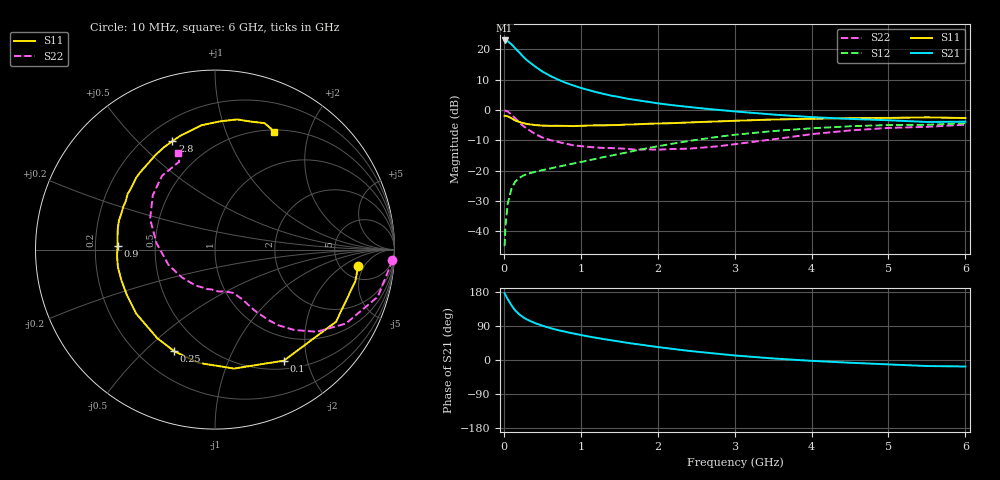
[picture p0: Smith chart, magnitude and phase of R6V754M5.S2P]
! SIEMENS Small Signal Semiconductors
! BFR193
! Si NPN RF Bipolar Junction Transistor in SOT23
! VCE = 0.75 V  IC = 4.5 mA
! Common Emitter S-Parameters:  May  1996
# GHz  S  MA  R  50
!  f  S11  S21  S12  S22
! GHz  MAG  ANG  MAG  ANG  MAG  ANG  MAG  ANG
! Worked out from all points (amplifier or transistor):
!   36 points, 10 MHz to 6 GHz, reference 50 ohm
!   highest |S21| = 22.9 dB at 10 MHz (marker M1)
!   |S21| within 3 dB of that: start of sweep to 164.5 MHz
!   unconditionally stable (mu >= 1): 883.6 MHz to 2.277 GHz
!   at 250 MHz: K = 0.41, MSG = 19.6 dB, |S12| = -21.6 dB
!   at 1.4 GHz: K = 1.09, MAG = 8.0 dB, |S12| = -15.0 dB
!   at 6 GHz: K = 1.00, MSG = 0.3 dB, |S12| = -4.4 dB
!   S11 on the Smith chart (normalised r, x): 10 MHz: 7.28, -3.67; 100 MHz: 0.62, -1.62; 250 MHz: 0.34, -0.62; 900 MHz: 0.30, +0.02; 2.8 GHz: 0.30, +0.64; 6 GHz: 0.52, +1.49
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0.01  0.8031 -6.4  14 176.3  0.0057 87.1  0.9891 -3.3
0.02  0.8016 -12.6  13.86 172.0  0.0117 85.6  0.975 -6.5
0.05  0.7851 -30.8  13.64 160.6  0.0285 75.1  0.9438 -16.2
0.1  0.728 -58.2  12.07 144.1  0.051 62.8  0.8374 -29.5
0.15  0.6712 -80.9  10.35 130.3  0.0666 53.6  0.7288 -38.9
0.2  0.6376 -98.3  8.914 120.6  0.0758 48.0  0.6277 -45.5
0.25  0.6099 -112.0  7.595 113.0  0.0829 44.5  0.5493 -50.1
0.3  0.5889 -123.2  6.628 106.9  0.0881 42.7  0.4944 -52.7
0.4  0.5658 -140.9  5.28 97.8  0.0952 41.0  0.4081 -56.8
0.5  0.5529 -152.2  4.317 90.5  0.102 41.2  0.3518 -59.3
0.6  0.549 -161.7  3.662 84.5  0.1087 42.2  0.3204 -60.9
0.7  0.5496 -169.6  3.195 79.1  0.1157 43.5  0.2983 -62.8
0.9  0.5434 177.9  2.546 70.1  0.1308 46.6  0.2627 -67.2
1.1  0.5546 167.5  2.134 62.1  0.1479 49.0  0.247 -73.0
1.3  0.5593 159.0  1.838 55.1  0.1677 50.6  0.2368 -78.9
1.6  0.5769 147.6  1.539 45.5  0.2003 51.7  0.2293 -90.2
2.2  0.6075 128.1  1.198 29.2  0.2793 49.3  0.2277 -118.1
2.8  0.6496 111.4  1.001 16.0  0.3634 42.3  0.2535 -152.0
3.5  0.6969 96.2  0.842 4.1  0.4495 31.2  0.3284 173.5
4.5  0.7358 80.3  0.713 -7.2  0.5397 15.0  0.4605 138.8
5.5  0.7567 68.6  0.635 -15.9  0.5709 -0.4  0.5281 112.3
6  0.7365 63.3  0.642 -17.1  0.6037 -5.0  0.5735 110.8
